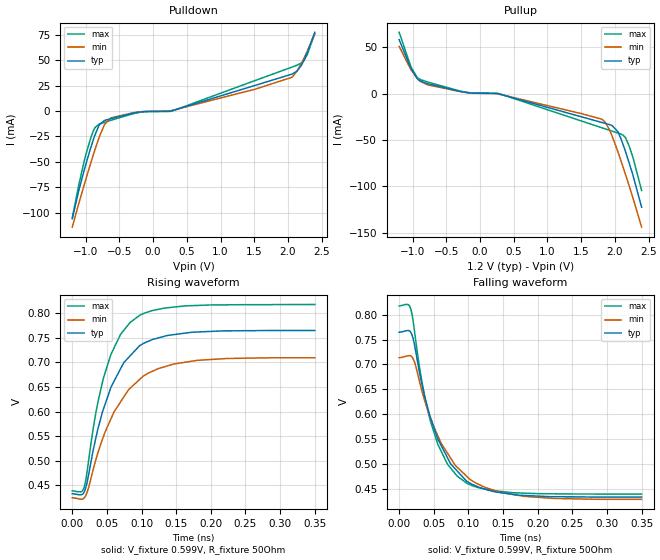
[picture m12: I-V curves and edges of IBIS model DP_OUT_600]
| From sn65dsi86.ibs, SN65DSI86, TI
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|   Model
[Model]   DP_OUT_600
Model_type   Output
Polarity   Non-Inverting
Vmeas = 0.6
Vref = 0.6
Cref = 1pF
Rref = 50
|   typ   min   max
C_comp   0.503pF   0.476pF   0.611pF
[Voltage Range]   1.2   1.14   1.26
[Temperature Range]   27   125   -40
[Pullup Reference]   1.2   1.14   1.26
[Pulldown Reference]   -0   -0   -0
[Power Clamp Reference]   1.2   1.14   1.26
[GND Clamp Reference]   -0   -0   -0
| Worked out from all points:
|   slope of the pulldown table from 0 to 0.18 V, typ, clamps not added: 1.96 kohm
|   slope of the pullup table from 0 to 0.18 V, typ, clamps not added: 1.89 kohm
|   falling waveform, V_fixture 0.599V, R_fixture 50Ohm: 20-80 % time 47.1ps typ, 58.4ps min, 39.8ps max; typ from 0.765 V to 0.433 V
|   rising waveform, V_fixture 0.599V, R_fixture 50Ohm: 20-80 % time 46.7ps typ, 57.3ps min, 39.6ps max; typ from 0.433 V to 0.765 V
[Pulldown]
|   Voltage   I(typ)   I(min)   I(max)
-1.2V     -106.1mA   -114.4mA   -105.2mA
-1.024V   -58.39mA   -72.81mA   -49.53mA
-897.6mV  -30.29mA   -45.21mA   -21.31mA
-789.6mV  -12.8mA    -23.91mA   -12.75mA
-717.6mV  -9.3mA     -12.94mA   -11.13mA
-624mV    -7.491mA   -6.713mA   -9.107mA
-177.6mV  -889.6uA   -761.3uA   -1.146mA
268.8mV   65.01uA    335.6uA    -251uA
2.058V    36.29mA    33.13mA    43.18mA
2.134V    39.3mA     39.35mA    45.06mA
2.238V    50.23mA    52.09mA    49.81mA
2.396V    77.42mA    75.87mA    76.32mA
[Pullup]
|   Voltage   I(typ)   I(min)   I(max)
-1.2V     58.26mA    50.99mA    66.15mA
-1.016V   26.19mA    24.93mA    27.78mA
-933.6mV  16.64mA    16.5mA     17.65mA
-886.8mV  13.75mA    13.33mA    15.35mA
-202.8mV  1.331mA    1.285mA    1.477mA
268.8mV   -25.16uA   -298.3uA   293.4uA
1.813V    -31.15mA   -27.72mA   -36.9mA
1.925V    -33.44mA   -39.75mA   -39.58mA
2.044V    -40.94mA   -62.41mA   -42.44mA
2.159V    -62.76mA   -87.41mA   -47.73mA
2.267V    -87.68mA   -112.1mA   -68.47mA
2.396V    -122.4mA   -143.9mA   -104.4mA
[Ramp]
R_load = 50
|   typ   min   max
dV/dt_r   0.199049/4.67228e-11   0.170731/5.72672e-11   0.227276/3.96199e-11
dV/dt_f   0.199049/4.71417e-11   0.17104/5.84011e-11   0.227276/3.98465e-11
[Falling Waveform]
V_fixture = 0.599V
V_fixture_min = 0.569V
V_fixture_max = 0.628V
R_fixture = 50Ohm
C_fixture = 0F
|   Time   V(typ)   V(min)   V(max)
0s        764.8mV    713.5mV    817.7mV
16.9ps    764.3mV    717mV      811.3mV
22.15ps   739.4mV    705mV      767mV
33.05ps   659.1mV    645.8mV    663.4mV
44.82ps   595mV      593.4mV    587.2mV
55.84ps   549.9mV    556.3mV    539mV
83.6ps    485.8mV    493.3mV    475.3mV
105.3ps   458.7mV    465.8mV    456.1mV
146.3ps   442mV      442.6mV    444.4mV
350ps     433.1mV    428.5mV    438.9mV
[Rising Waveform]
V_fixture = 0.599V
V_fixture_min = 0.569V
V_fixture_max = 0.628V
R_fixture = 50Ohm
C_fixture = 0F
|   Time   V(typ)   V(min)   V(max)
0s        433.1mV    424.9mV    438.9mV
16.9ps    436mV      423.9mV    445mV
22.15ps   461.3mV    438.8mV    485.6mV
33.05ps   540.4mV    497.1mV    589.6mV
44.82ps   604.4mV    548.6mV    667.3mV
55.84ps   649.5mV    585.3mV    716.5mV
83.6ps    713.5mV    647.5mV    781.4mV
105.3ps   740.3mV    674.4mV    800.7mV
146.3ps   756.4mV    696.7mV    812.4mV
350ps     764.8mV    709.4mV    817.7mV
